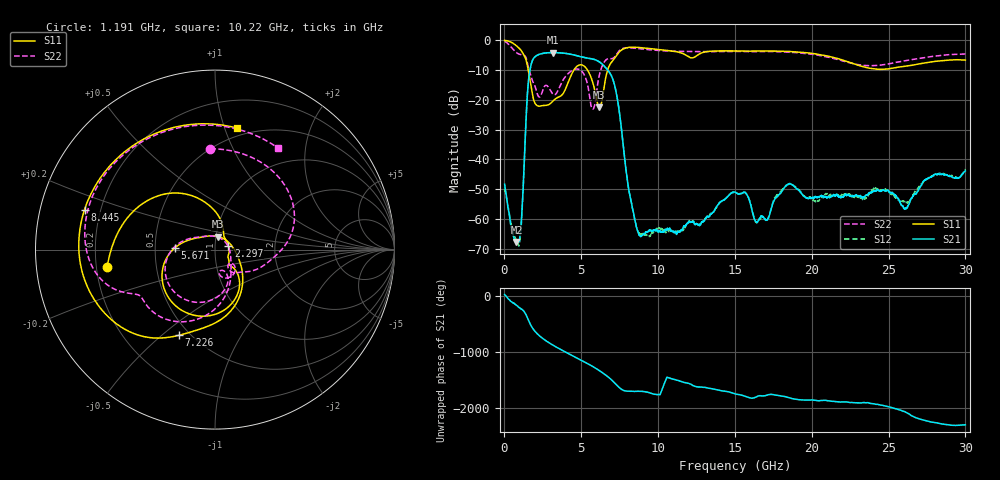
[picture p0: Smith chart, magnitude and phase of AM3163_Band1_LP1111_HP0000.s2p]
!Agilent Technologies,E8364B,MY43040894,A.07.50.67
!Agilent E8364B: A.07.50.67
!Date: Thursday, August 20, 2020 11:29:54
!Correction: S11(Full 2 Port(1,2))
!S21(Full 2 Port(1,2))
!S12(Full 2 Port(1,2))
!S22(Full 2 Port(1,2))
!S2P File: Measurements: S11, S21, S12, S22:
# Hz S  dB  R 50
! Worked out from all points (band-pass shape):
!   3201 points, 10 MHz to 30 GHz, reference 50 ohm
!   highest |S21| = -4.18 dB at 3.178 GHz (marker M1); lowest = -67.8 dB at 778.5 MHz (marker M2)
!   |S21| within 3 dB of the highest: 1.794 GHz to 6.144 GHz (4.349 GHz wide, 110 % of centre)
!   lowest |S11| = -22.5 dB at 6.177 GHz (marker M3), VSWR 1.16, Z = 51.2 + j7.5 ohm
!   |S11| at or under -10 dB: 1.546 GHz to 4.526 GHz (2.98 GHz wide, 98.2 % of centre); 5.4 GHz to 6.717 GHz (1.317 GHz wide, 21.7 % of centre)
!   |S22| runs from -23.2 to -0.4 dB; largest |S21 - S12| = 0.0062
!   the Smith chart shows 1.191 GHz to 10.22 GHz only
!   S11 on the Smith chart (normalised r, x): 1.191 GHz: 0.25, -0.07; 2.297 GHz: 1.16, +0.05; 5.671 GHz: 0.63, +0.01; 7.226 GHz: 0.44, -0.57; 8.445 GHz: 0.14, +0.15; 10.22 GHz: 0.43, +1.10
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1e7  -0.10 -8.8  -48.37 25.3  -49.85 -97.1  -0.38 -15.5
3.942469e8  -0.59 -52.3  -61.62 -92.3  -60.69 -87.0  -2.11 -86.9
7.784938e8  -1.88 -104.9  -67.79 -164.4  -67.06 64.0  -4.15 -168.5
1.190856e9  -4.32 -171.0  -52.44 108.2  -53.18 166.5  -5.00 92.7
1.612591e9  -11.98 98.2  -11.54 -106.7  -11.53 -106.8  -10.26 -12.6
1.996838e9  -21.26 53.0  -5.53 87.7  -5.54 87.7  -15.57 -50.9
2.296738e9  -22.17 17.0  -4.70 6.9  -4.71 6.9  -19.08 -45.0
2.727844e9  -21.88 -23.1  -4.27 -81.7  -4.28 -81.7  -15.18 -62.3
3.177694e9  -20.33 -36.8  -4.18 -158.3  -4.19 -158.2  -18.24 -77.0
3.946188e9  -16.72 -44.8  -4.41 86.0  -4.43 86.0  -12.37 -79.6
5.014581e9  -8.29 -120.5  -5.62 -65.1  -5.61 -64.9  -10.36 -156.2
5.670612e9  -13.01 177.4  -6.27 -161.5  -6.24 -161.5  -22.68 89.2
6.176694e9  -22.52 76.5  -7.29 112.3  -7.32 112.1  -11.71 -76.7
7.226344e9  -5.70 -112.9  -16.39 -122.4  -16.38 -121.8  -5.29 -153.6
8.444688e9  -2.38 162.9  -59.08 102.1  -59.37 99.5  -2.68 133.2
1.000979e10  -3.14 88.5  -64.16 45.2  -63.14 38.0  -3.45 66.0
1.021597e10  -3.25 79.7  -64.18 106.1  -63.19 23.3  -3.53 58.1
1.5005e10  -3.62 -71.5  -51.01 59.3  -51.17 60.6  -3.80 -91.9
2.000958e10  -4.43 163.2  -52.99 -50.5  -53.37 -48.9  -4.71 136.4
2.275554e10  -7.99 60.1  -52.28 -99.2  -52.60 -99.1  -7.97 20.7
2.500479e10  -9.64 -62.4  -50.67 -170.9  -50.74 -165.3  -7.97 -92.7
3e10  -6.70 104.3  -43.90 -131.9  -43.30 -130.3  -4.65 102.1
